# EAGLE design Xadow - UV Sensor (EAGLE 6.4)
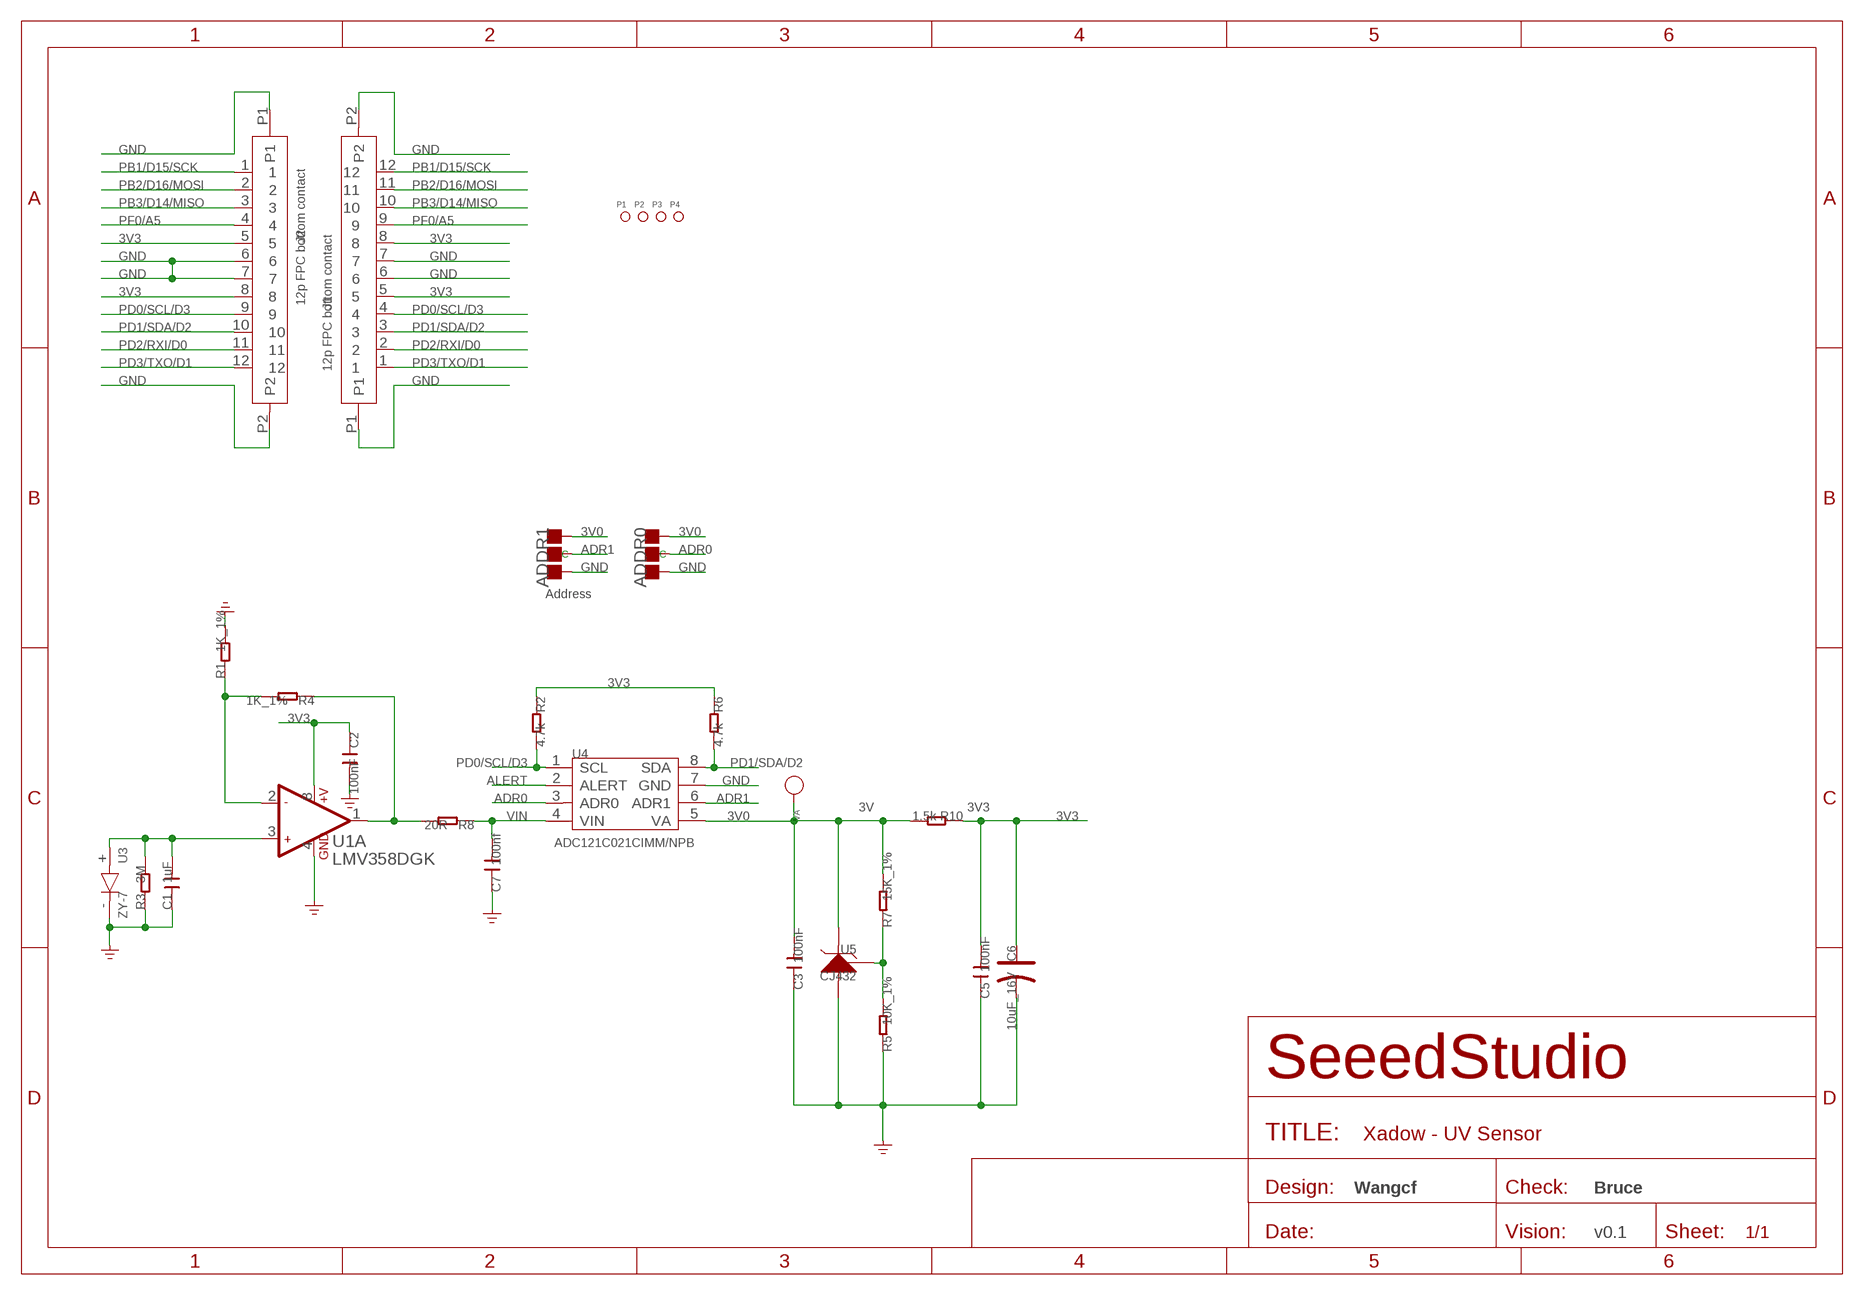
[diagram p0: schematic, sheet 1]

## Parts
ADDR0  DNP  PAD-JUMPER-3P-40*40  [3P-SMD-4.1X1.5]
ADDR1  DNP  PAD-JUMPER-3P-40*40  [3P-SMD-4.1X1.5]
C1  1uF  C-0805  [C0805]
C2  100nF  C-0603  [C0603]
C3  100nF  C-0603  [C0603]
C5  100nF  C-0603  [C0603]
C6  10uF_16V  CAP-AVX-A  [AVX-A]
C7  100nf  C-0603  [C0603]
J1  12p FPC bottom contact  FPC052002-12LT  [12P-0.5]
J2  12p FPC bottom contact  FPC052002-12LT  [12P-0.5]
P1  PAD-MARK  [ROUND-MARK-1.0]
P2  PAD-MARK  [ROUND-MARK-1.0]
P3  PAD-MARK  [ROUND-MARK-1.0]
P4  PAD-MARK  [ROUND-MARK-1.0]
R1  1K_1%  R-0603  [R0603]
R2  4.7k  R-0603  [R0603]
R3  3M  R-0603  [R0603]
R4  1K_1%  R-0603  [R0603]
R5  10K_1%  R-0603  [R0603]
R6  4.7k  R-0603  [R0603]
R7  15K_1%  R-0603  [R0603]
R8  20R  R-0603  [R0603]
R10  1.5k  R-0603  [R0603]
U1  LMV358DGK  [MSOP8]
U3  ZY-7  TP-6  [2P-SMD-2X1.25]
U4  ADC121C021CIMM/NPB  ADC121C021'CIMM/NP8'  [MSOP8]
U5  CJ432  REFERENCE-SOURCE  [SOT23]
VA  DNP  PAD-TEST-POINT-CIRCLE'3535'  [TP_3535]

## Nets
3V0: ADDR0.11(R) ADDR1.11(R) C3.2 R7.2 R10.2 U4.5(VA) U5.2(K) VA.T
3V3: C2.1 C5.2 C6.+ J1.5 J1.8 J2.5 J2.8 R2.1 R6.1 R10.1 U1.8(A:+V)
ADR0: ADDR0.MM(C) U4.3(ADR0)
ADR1: ADDR1.MM(C) U4.6(ADR1)
ALERT: U4.2(ALERT)
GND: ADDR0.00(L) ADDR1.00(L) C1.1 C2.2 C3.1 C5.1 C6.- C7.1 J1.6 J1.7 J1.P1 J1.P2 J2.6 J2.7 J2.P1 J2.P2 R1.2 R3.1 R5.1 U1.4(A:GND) U3.- U4.7(GND) U5.3(A)
N$1: R5.2 R7.1 U5.1(R)
N$3: C1.2 R3.2 U1.3(A:+IN1) U3.+
N$5: R1.1 R4.2 U1.2(A:-IN1)
PB1/D15/SCK: J1.12 J2.1
PB2/D16/MOSI: J1.11 J2.2
PB3/D14/MISO: J1.10 J2.3
PD0/SCL/D3: J1.4 J2.9 R2.2 U4.1(SCL)
PD1/SDA/D2: J1.3 J2.10 R6.2 U4.8(SDA)
PD2/RXI/D0: J1.2 J2.11
PD3/TXO/D1: J1.1 J2.12
PF0/A5: J1.9 J2.4
SIG1: R4.1 R8.2 U1.1(A:OUT1)
VIN: C7.2 R8.1 U4.4(VIN)
Unconnected: U1.5(B:+IN2) U1.6(B:-IN2) U1.7(B:OUT2)

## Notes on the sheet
- Address
- 3V | 3V3
- Wangcf | Bruce
- v0.1

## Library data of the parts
ADDR0 ADDR1 = Discrete:PAD-JUMPER-3P; PARTNO: DNP
C1 = Discrete1:C*: Ceramic Capacitors
C2 = Discrete (1):C*: Ceramic Capacitors
C3 C5 C7 = Discrete:C*: Ceramic Capacitors
C6 = Discrete1:CAP*: Electrolytic Capacitors,Tantalum Capacitors and Super Capacitors
J1 J2 = template:FPC052002-12LT
P1-P4 = Discrete:PAD-MARK; PARTNO: DNP
R1-R8 R10 = Discrete:R*
U1 = IC:LMV358: General purpose LOW Voltage, Rail-to-Rail Output Amplifiers http://www.fairchildsemi.com/ds/LM/LMV358.pdf
U3 = template:TP-6
U4 = IC:ADC121C021: ADC121C021/ADC121C021Q/ADC121C027 I2C-Compatible, 12-Bit Analog-to-Digital Converter with Alert Function
U5 = For_Test_Albert_v6:REFERENCE-SOURCE: CJ432,AZ432 or other Adjustable Reference Source
VA = Discrete:PAD-TEST-POINT-CIRCLE; PARTNO: DNP

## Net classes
1 GND: width 0.152 mm, drill 0.305 mm, clearance 0.152 mm to class 0, clearance 0.152 mm
3 usbvcc: width 0.203 mm, drill 0.305 mm, clearance 0.203 mm

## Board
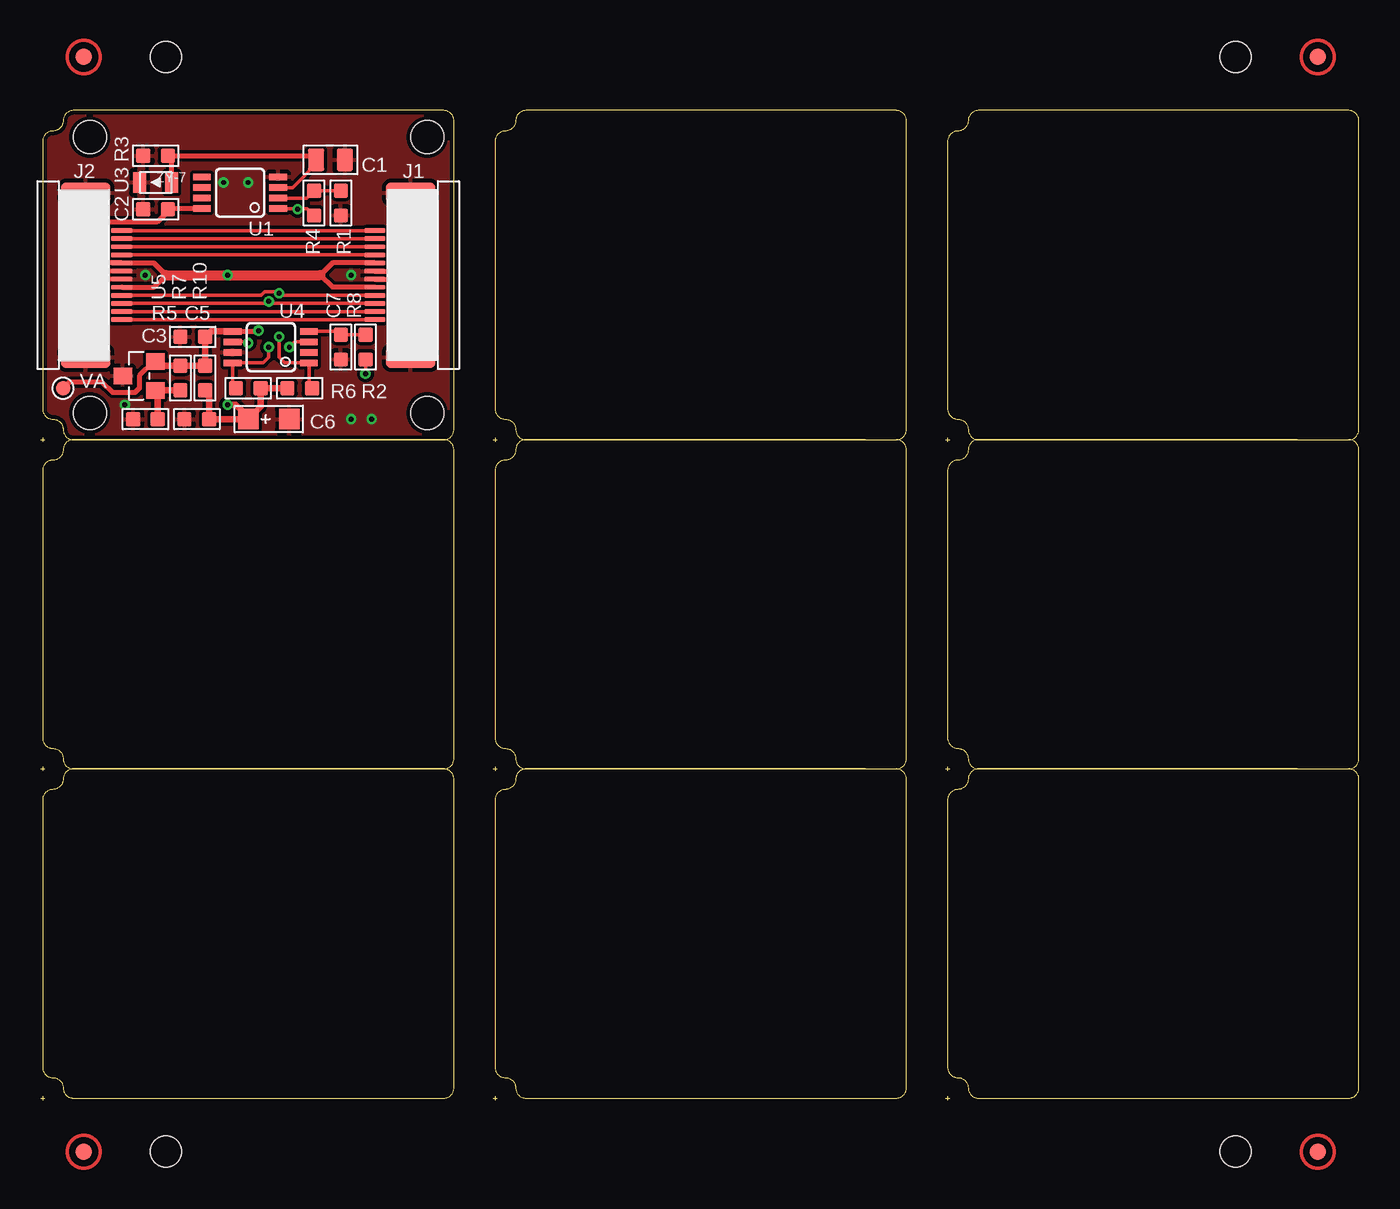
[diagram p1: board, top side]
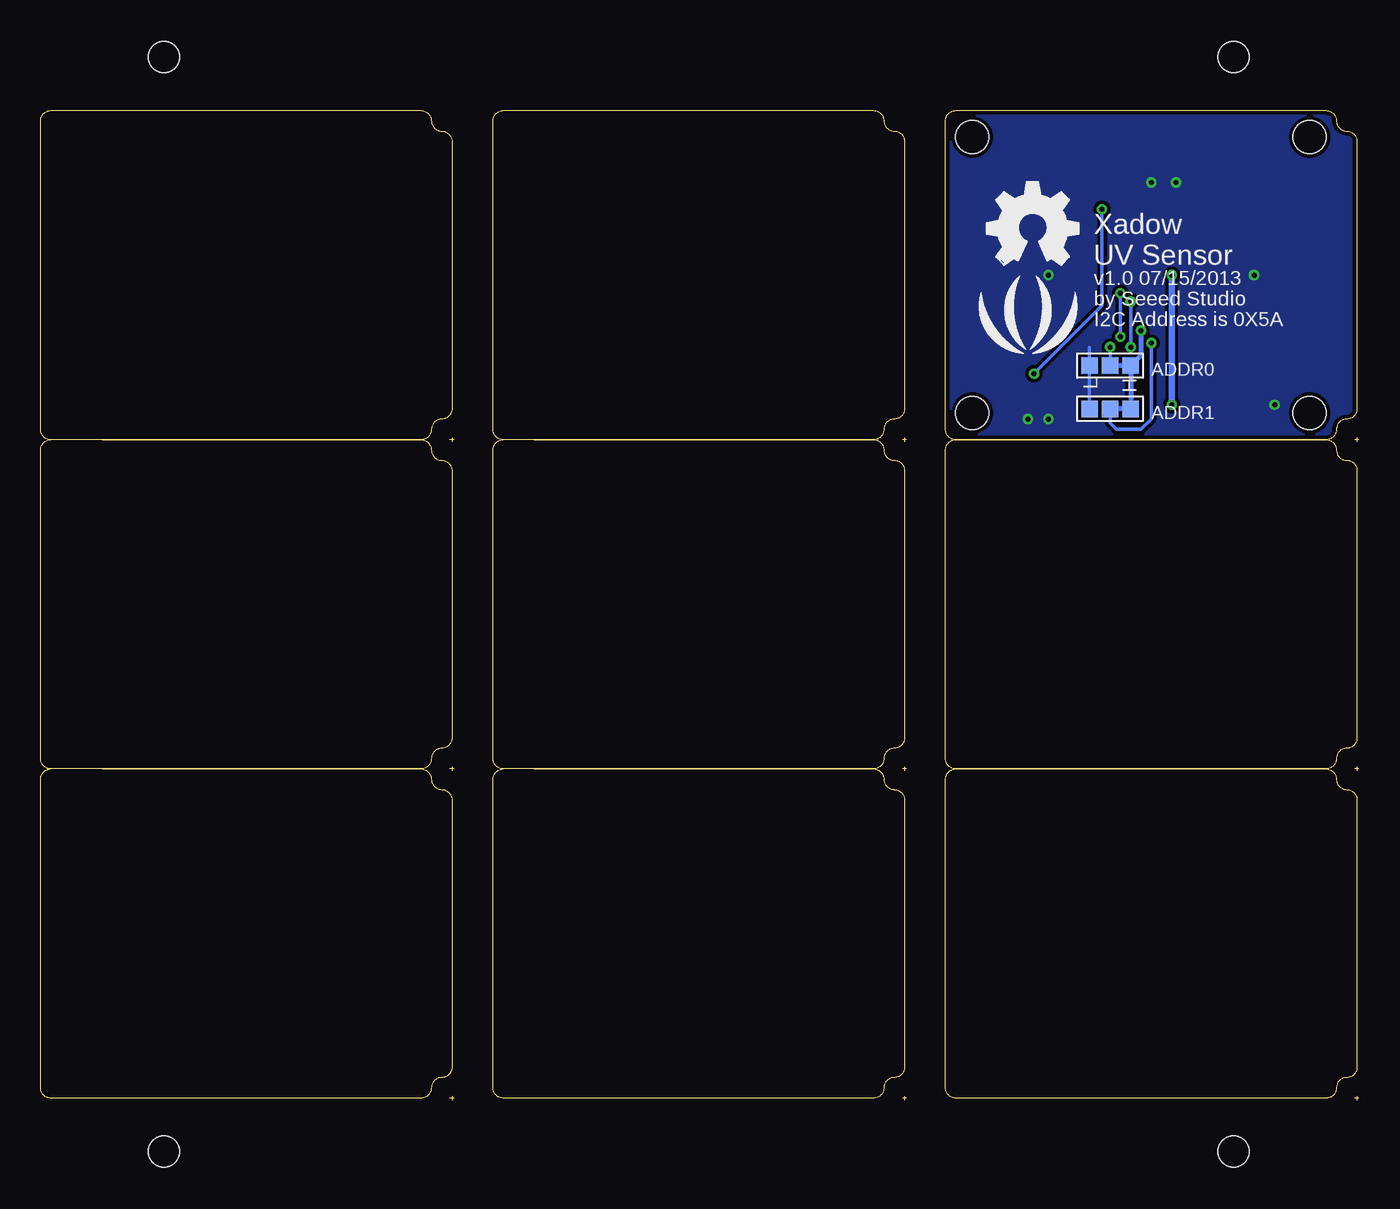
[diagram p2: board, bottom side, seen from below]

Size 81.41 x 61.09 mm. Coordinates in mm from the lower left corner, seen from the top.
Outline: 173 segments
Copper layers (1*16): Top 0.035mm / dielectric 1.5mm / Bottom 0.035mm
Design rules "SeeedStudio_rule_no_angle_090911 *": minimum track width 6mil, minimum drill 12mil, track to track 6mil, track to pad 6mil, pad to pad 6mil, via to via 6mil, smd to smd 0mil, copper to edge 10mil, drill to drill 10mil, minimum pad ring 10mil, minimum via ring 6mil, stop-mask expansion 2mil, vias tented up to drill 25mil, thermal gap 10mil
Holes 2.03 mm at 3.05,42.42 3.05,59.44 23.88,59.44 23.88,42.42
Holes 1.91 mm at 73.79,64.39 7.75,64.39 7.75,-3.17 73.79,-3.17
tRestrict: area 20.3,50.7 to 21,51.2; area 4.8,50.7 to 5.3,51.2

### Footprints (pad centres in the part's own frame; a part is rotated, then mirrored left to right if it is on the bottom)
3P-SMD-4.1X1.5 = smd 1.016 x 1.016: 00 -1.27,0; 11 1.27,0; MM 0,0
C0805 = smd 1.016 x 1.397: 1 -0.889,0; 2 0.889,0
C0603 = smd 0.889 x 0.889: 1 -0.762,0; 2 0.762,0
AVX-A = smd 1.27 x 1.27: + -1.27,0; - 1.27,0
12P-0.5 = smd 0.3 x 1.3: 1 -2.75,2.35; 2 -2.25,2.35; 3 -1.75,2.35; 4 -1.25,2.35; 5 -0.75,2.35; 6 -0.25,2.35; 7 0.25,2.35; 8 0.75,2.35; 9 1.25,2.35; 10 1.75,2.35; 11 2.25,2.35; 12 2.75,2.35 | smd 1.27 x 3.048: P1 -5.08,0.127; P2 5.08,0.127
ROUND-MARK-1.0 = smd 1.016 x 1.016: P$1 0,0
R0603 = smd 0.889 x 0.889: 1 -0.762,0; 2 0.762,0
MSOP8 = smd 1.1 x 0.4: 1 -2.477,0.975; 2 -2.477,0.325; 3 -2.477,-0.325; 4 -2.477,-0.975; 5 2.223,-0.975; 6 2.223,-0.325; 7 2.223,0.325; 8 2.223,0.975
2P-SMD-2X1.25 = smd 0.8 x 1.27: + -1,0; - 1,0
SOT23 = smd 1.016 x 1.143: 1 -0.889,-1.016; 2 0.889,-1.016; 3 0,1.016
TP_3535 = smd 0.889 x 0.889: T 0,0

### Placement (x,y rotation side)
ADDR0  15.37,45.34 0 bottom
ADDR1  15.37,42.67 0 bottom
C1  17.91,58.04 180 top
C2  7.11,54.99 180 top
C3  9.4,47.12 0 top
C5  9.65,42.04 0 top
C6  14.1,42.04 0 top
C7  18.54,46.48 90 top
J1  22.99,50.93 90 top
J2  2.67,50.93 270 top
P1  not placed on the board
P2  not placed on the board
P3  not placed on the board
P4  not placed on the board
R1  18.54,55.37 270 top
R2  16,43.94 0 top
R3  7.11,58.29 0 top
R4  16.89,55.37 90 top
R5  6.48,42.04 0 top
R6  12.83,43.94 180 top
R7  8.64,44.58 90 top
R8  20.07,46.48 270 top
R10  10.16,44.58 90 top
U1  12.19,56.01 180 top
U3  7.11,56.64 180 top
U4  14.1,46.48 180 top
U5  6.1,44.7 90 top
U$2  [LOGO_SILK]  20.45,47.75 0 bottom
U$3  [OSHW_FILLX200_NOTEXT]  22.99,51.56 0 bottom
VA  1.4,43.94 270 top

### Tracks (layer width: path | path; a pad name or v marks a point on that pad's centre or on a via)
3V0  (via drill 0.3 pad 0.64)
  Top 0.305: U4.5 13.42,47.46 v13.46,47.5 | U5.2 6.99,45.59 6.1,44.7 6.1,43.94 5.84,43.69 4.45,43.69 3.81,44.32 1.78,44.32 VA.T 1.4,44.2
  Top 0.406: R10.2 10.03,45.34 | 10.03,45.34 R7.2 7.37,45.34 U5.2 | U4.5 10.5,47.46 C3.2 10.16,45.47 10.03,45.34
  Bottom 0.305: ADDR0.11 ADDR1.11 15.37,42.67 | v13.46,47.5 13.46,45.97 ADDR0.11 | ADDR0.11 15.37,45.34
3V3  (via drill 0.3 pad 0.64)
  Top 0.305: J2.8 7,50.18 7.75,50.93 7,51.68 J2.5 3.95,51.68 3.56,52.07 3.56,53.85 3.94,54.23 7.22,54.23 8.03,55.03 | J1.8 18.02,51.68 17.27,50.93 18.02,50.18 J1.5 | U1.8 8.03,55.03 | 8.03,55.03 7.92,55.03 C2.1
  Top 0.406: R10.1 10.29,43.81 10.41,43.69 C5.2 C6.+ | C6.+ 13.59,42.8 R6.1 R2.1 | v11.56,42.93 12.06,42.93 12.57,42.42 12.57,42.29 C6.+
  Top 0.61: 7.75,50.93 v11.56,50.93 17.27,50.93
  Bottom 0.406: v11.56,42.93 v11.56,50.93
ADR0  (via drill 0.3 pad 0.64)
  Top 0.203: U4.3 15.69,46.81 v15.37,46.48
  Bottom 0.203: v15.37,46.48 ADDR0.MM
ADR1  (via drill 0.3 pad 0.64)
  Top 0.203: U4.6 12.76,46.81 v12.83,46.74
  Bottom 0.203: v12.83,46.74 12.83,42.04 13.46,41.4 14.99,41.4 15.37,41.78 ADDR1.MM
GND  (via drill 0.3 pad 0.64)
  Top 0.305: J2.6 3.05,51.18 | J2.7 3.05,50.68 3.05,50.67 | J1.7 22.73,51.18 | J1.6 22.73,50.68 22.73,50.67
  Bottom 0.203: ADDR0.00 ADDR1.00 16.64,46.48
  other vias: 6.48,50.93 19.18,42.04 20.45,42.04 19.18,50.93 5.21,42.93 12.83,56.64 11.3,56.64
  pour Top (isolate 0.203): 0.13,40.77 25.53,40.77 25.53,61.09 0.13,61.09
  pour Bottom (isolate 0.203): 0.13,40.77 25.53,40.77 25.53,61.09 0.13,61.09
N$1
  Top 0.406: U5.1 7.24,43.81 | 7.24,43.81 R7.1 | R5.2 7.24,43.81
N$3
  Top 0.203: U1.3 15.56,56.33 17.14,57.91 C1.2
  Top 0.305: U3.+ 8.11,58.28 | 8.11,58.28 8.13,58.29 | R3.2 8,58.29 | 8,58.29 16.76,58.29 C1.2 | 8.11,58.28 8.02,58.28 8,58.29
N$5
  Top 0.203: R1.1 R4.2 16.44,55.68 U1.2
PB1/D15/SCK
  Top 0.203: J1.12 J2.1
PB2/D16/MOSI
  Top 0.203: J2.2 J1.11
PB3/D14/MISO
  Top 0.203: J1.10 J2.3
PD0/SCL/D3  (via drill 0.3 pad 0.64)
  Top 0.203: R2.2 16.57,44.13 U4.1 15.07,45.51 14.73,45.85 v14.73,47.12 | J2.9 13.61,49.68 13.84,49.91 14.61,49.91 14.73,49.78 | J1.4 14.84,49.68 14.73,49.78 | v14.73,49.8 14.73,49.78
  Bottom 0.203: v14.73,47.12 v14.73,49.8
PD1/SDA/D2  (via drill 0.3 pad 0.64)
  Top 0.203: R6.2 11.87,44.13 U4.8 13.76,45.51 14.1,45.85 v14.1,46.48 | J2.10 14.1,49.18 | 14.1,49.18 J1.3 | v14.1,49.3 14.1,49.18
  Bottom 0.203: v14.1,46.48 v14.1,49.3
PD2/RXI/D0
  Top 0.203: J1.2 J2.11
PD3/TXO/D1
  Top 0.203: J2.12 J1.1
PF0/A5
  Top 0.203: J2.4 J1.9
SIG1  (via drill 0.3 pad 0.64)
  Top 0.203: R8.2 v20.07,44.83 | U1.1 15.92,55.03 | R4.1 16.47,55.03 15.92,55.03 | 15.92,55.03 v15.88,54.99
  Bottom 0.203: v20.07,44.83 15.88,49.02 v15.88,54.99
VIN
  Top 0.203: R8.1 C7.2 18.33,47.46 U4.4

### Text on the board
bPlace: Xadow | UV Sensor | v1.0 07/15/2013 | by Seeed Studio | I2C Address is 0X5A | H | L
